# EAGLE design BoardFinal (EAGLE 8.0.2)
two capacitors for regulator (in & out) 10uF each
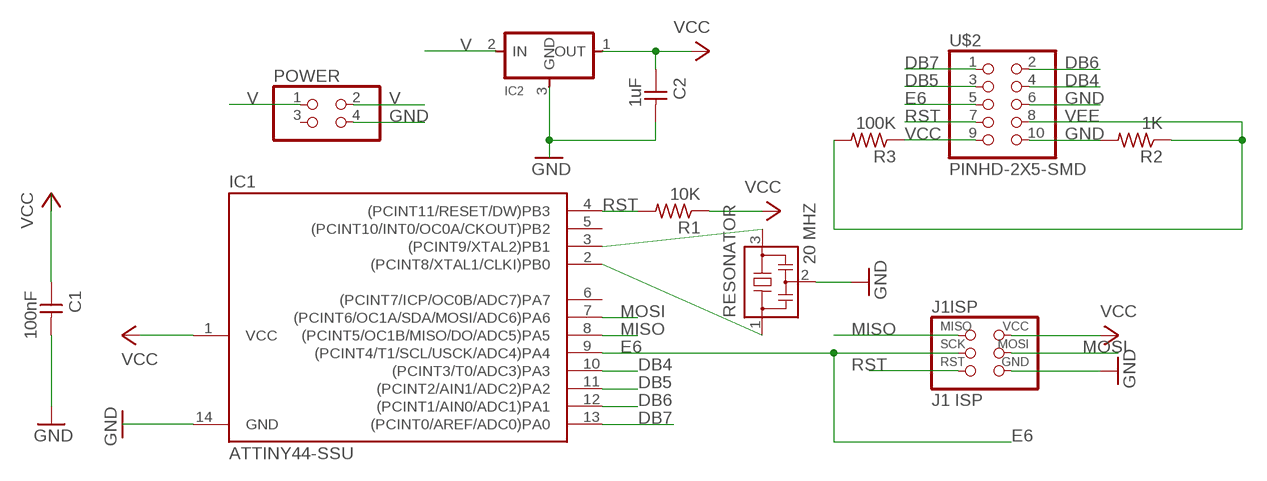
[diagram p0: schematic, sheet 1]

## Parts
C1  100nF  CAP-UNPOLARIZEDFAB  [C1206FAB]
C2  1uF  CAP-UNPOLARIZEDFAB  [C1206FAB]
IC1  ATTINY44-SSU  [SOIC14]
IC2  REGULATORSOT23  [SOT23]
J1ISP  J1 ISP  AVRISPSMD  [2X03SMD]
POWER  PINHD-2X2-SMD  [2X02SMD]
R1  10K  RES-US1206FAB  [R1206FAB]
R2  1K  RES-US1206FAB  [R1206FAB]
R3  100K  RES-US1206FAB  [R1206FAB]
RESONATOR  20 MHZ  RESONATOR  [EFOBM]
U$2  PINHD-2X5-SMD  [2X05SMD]

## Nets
DB4: IC1.10((PCINT3/T0/ADC3)PA3) U$2.4
DB5: IC1.11((PCINT2/AIN1/ADC2)PA2) U$2.3
DB6: IC1.12((PCINT1/AIN0/ADC1)PA1) U$2.2
DB7: IC1.13((PCINT0/AREF/ADC0)PA0) U$2.1
E6: IC1.9((PCINT4/T1/SCL/USCK/ADC4)PA4) J1ISP.3(SCK) U$2.5
GND: C1.2 C2.2 IC1.14(GND) IC2.3(GND) J1ISP.6(GND) POWER.4 R2.2 RESONATOR.2 U$2.6 U$2.10
MISO: IC1.8((PCINT5/OC1B/MISO/DO/ADC5)PA5) J1ISP.1(MISO)
MOSI: IC1.7((PCINT6/OC1A/SDA/MOSI/ADC6)PA6) J1ISP.4(MOSI)
N$2: IC1.2((PCINT8/XTAL1/CLKI)PB0) RESONATOR.1
N$3: IC1.3((PCINT9/XTAL2)PB1) RESONATOR.3
RST: IC1.4((PCINT11/RESET/DW)PB3) J1ISP.5(RST) R1.2 U$2.7
V: IC2.2(IN) POWER.1 POWER.2
VCC: C1.1 C2.1 IC1.1(VCC) IC2.1(OUT) J1ISP.2(VCC) R1.1 R3.1 U$2.9
VEE: R2.1 R3.2 U$2.8
Unconnected: IC1.5((PCINT10/INT0/OC0A/CKOUT)PB2) IC1.6((PCINT7/ICP/OC0B/ADC7)PA7) POWER.3

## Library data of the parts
C1 C2 = fab:CAP-UNPOLARIZED
IC1 = fab:ATTINY44
IC2 = fab:REGULATOR
J1ISP = fab:AVRISP
POWER = fab:PINHD-2X2-SMD
R1-R3 = fab:RES-US: Resistor (US Symbol)
RESONATOR = fab:RESONATOR
U$2 = fab:PINHD-2X5-SMD

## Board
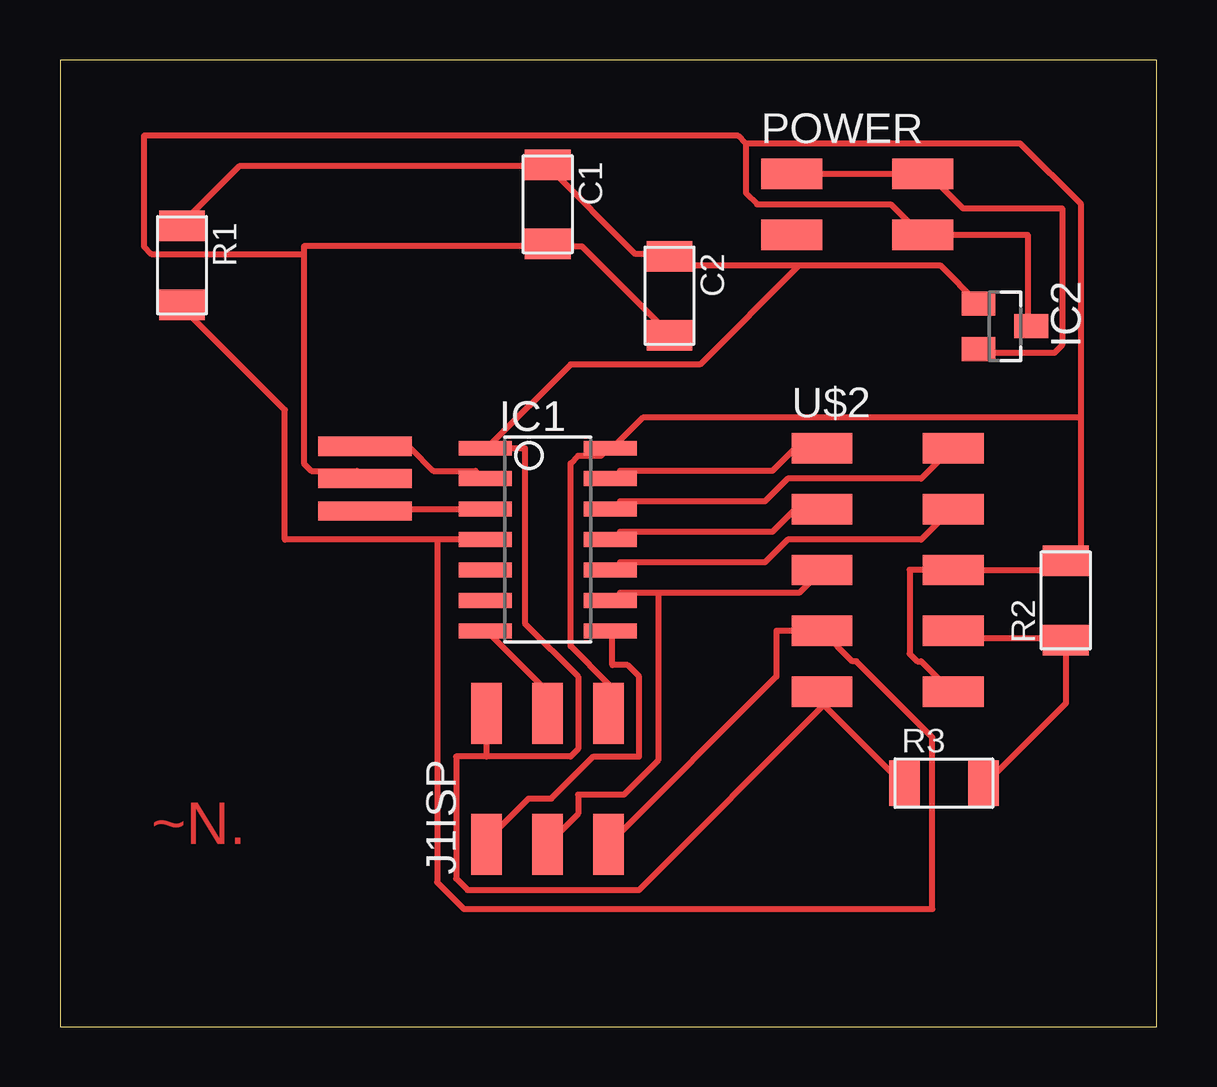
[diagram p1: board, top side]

Size 45.7 x 40.31 mm. Coordinates in mm from the lower left corner, seen from the top.
Outline: 0,0 45.7,0 45.7,40.31 0,40.31 0,0
Copper layers (1*16): Top 0.035mm / dielectric 1.5mm / Bottom 0.035mm
Design rules "default *": minimum track width 10mil, minimum drill 24mil, track to track 16mil, track to pad 16mil, pad to pad 16mil, via to via 16mil, smd to smd 8mil, copper to edge 40mil, drill to drill 8mil, minimum pad ring 10mil, minimum via ring 8mil, stop-mask expansion 4mil, vias tented up to drill 0mil, thermal gap 10mil

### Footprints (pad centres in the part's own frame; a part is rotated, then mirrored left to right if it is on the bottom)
C1206FAB = smd 1.27 x 1.905: 1 -1.651,0; 2 1.651,0
SOIC14 = smd 0.61 x 2.21: 1 -3.81,-2.603; 2 -2.54,-2.603; 3 -1.27,-2.603; 4 0,-2.603; 5 1.27,-2.603; 6 2.54,-2.603; 7 3.81,-2.603; 8 3.81,2.603; 9 2.54,2.603; 10 1.27,2.603; 11 0,2.603; 12 -1.27,2.603; 13 -2.54,2.603; 14 -3.81,2.603
SOT23 = smd 1 x 1.4: 1 -0.95,-1.1; 2 0.95,-1.1; 3 0,1.1
2X03SMD = smd 2.54 x 1.27: 1 -2.54,2.54; 2 2.92,2.54; 3 -2.54,0; 4 2.92,0; 5 -2.54,-2.54; 6 2.92,-2.54
2X02SMD = smd 2.54 x 1.27: 1 -2.54,1.27; 2 2.92,1.27; 3 -2.54,-1.27; 4 2.92,-1.27
R1206FAB = smd 1.27 x 1.905: 1 -1.651,0; 2 1.651,0
EFOBM = smd 0.8 x 3.9: 1 -1.35,0; 2 0,0; 3 1.35,0
2X05SMD = smd 2.54 x 1.27: 1 -2.54,2.54; 2 2.92,2.54; 3 -2.54,0; 4 2.92,0; 5 -2.54,-2.54; 6 2.92,-2.54; 7 -2.54,-5.08; 8 2.92,-5.08; 9 -2.54,-7.62; 10 2.92,-7.62

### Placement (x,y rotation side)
C1  20.32,34.29 270 top
C2  25.4,30.48 270 top
IC1  20.32,20.32 270 top
IC2  39.37,29.21 270 top
J1ISP  20.32,10.16 90 top
POWER  33.02,34.29 0 top
R1  5.08,31.75 270 top
R2  41.91,17.78 90 top
R3  36.83,10.16 0 top
RESONATOR  12.7,22.86 270 top
U$2  34.29,21.59 0 top

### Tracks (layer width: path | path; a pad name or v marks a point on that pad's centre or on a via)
DB4
  Top 0.254: IC1.10 23.02,19.05 23.34,19.37 29.37,19.37 30.32,20.32 35.88,20.32 37.15,21.59 U$2.4
DB5
  Top 0.254: U$2.3 30.64,21.59 29.69,20.64 23.34,20.64 23.02,20.32 IC1.11
DB6
  Top 0.254: IC1.12 23.02,21.59 23.34,21.91 29.37,21.91 30.32,22.86 35.88,22.86 37.15,24.13 U$2.2
DB7
  Top 0.254: U$2.1 30.64,24.13 29.69,23.18 23.34,23.18 23.02,22.86 IC1.13
E6
  Top 0.254: 24.92,18.1 30.8,18.1 U$2.5 | 24.92,18.1 23.34,18.1 23.02,17.78 IC1.9 | J1ISP.3 21.59,8.89 21.59,9.68 23.5,9.68 24.92,11.11 24.92,18.1
GND
  Top 0.254: 20.32,32.54 21.75,32.54 25.4,28.89 C2.2 | RESONATOR.2 12.38,23.18 10.48,23.18 10.16,23.5 10.16,32.23 | 10.16,32.23 10.16,32.54 20.32,32.54 | 20.32,32.54 C1.2 | J1ISP.6 22.86,14.29 21.27,15.88 21.27,23.5 21.59,23.81 22.54,23.81 22.86,24.13 IC1.14 23.02,24.13 24.29,25.4 42.55,25.4 | IC2.3 40.32,29.21 40.32,33.02 POWER.4 35.88,33.02 34.61,34.29 29.05,34.29 28.57,34.77 28.57,36.83 | U$2.10 37.15,13.97 35.88,15.24 35.72,15.24 35.4,15.56 35.4,19.05 U$2.6 41.59,19.05 41.91,19.37 R2.2 41.91,19.53 42.55,19.53 42.55,25.4 | 28.57,36.83 40.01,36.83 42.55,34.29 42.55,25.4 | 10.16,32.23 3.81,32.23 3.49,32.54 3.49,37.15 28.26,37.15 28.57,36.83
MISO
  Top 0.254: J1ISP.1 17.78,7.78 19.53,9.53 20.48,9.53 22.23,11.27 24.13,11.27 24.13,14.61 23.65,15.08 23.02,15.08 23.02,16.51 IC1.8
MOSI
  Top 0.254: J1ISP.4 20.32,13.97 17.78,16.51 IC1.7
N$2
  Top 0.254: IC1.2 17.62,22.86 17.3,23.18 15.56,23.18 14.61,24.13 12.7,24.13 RESONATOR.1
N$3
  Top 0.254: IC1.3 12.7,21.59 RESONATOR.3
RST
  Top 0.254: J1ISP.5 29.84,14.61 29.84,16.51 U$2.7 33.02,15.24 33.18,15.24 36.35,12.06 36.35,4.92 16.83,4.92 15.72,6.03 15.72,20.32 | IC1.4 15.72,20.32 | 15.72,20.32 9.37,20.32 9.37,25.72 5.08,30 R1.2
V
  Top 0.254: IC2.2 38.42,28.26 38.58,28.1 41.43,28.1 41.75,28.42 41.75,34.13 37.62,34.13 36.2,35.56 POWER.2 POWER.1
VCC
  Top 0.254: 20.32,35.88 7.46,35.88 5.08,33.5 R1.1 | 31.83,13.41 31.75,13.49 U$2.9 | 31.83,13.41 35.08,10.16 R3.1 | 30.8,31.75 25.72,31.75 25.4,32.07 C2.1 25.4,32.23 23.97,32.23 20.32,35.88 | 30.8,31.75 36.67,31.75 IC2.1 | 30.8,31.75 26.67,27.62 21.27,27.62 17.78,24.13 IC1.1 19.37,24.13 19.37,16.83 21.59,14.61 21.59,11.59 21.27,11.27 17.78,11.27 | 17.78,11.27 J1ISP.2 | 31.83,13.41 24.13,5.71 16.99,5.71 16.51,6.19 16.51,11.27 17.78,11.27 | 20.32,35.88 C1.1
VEE
  Top 0.254: R3.2 38.58,10.16 41.91,13.49 R2.1 41.91,16.19 37.62,16.19 37.31,16.51 U$2.8

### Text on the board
Top: ~N.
